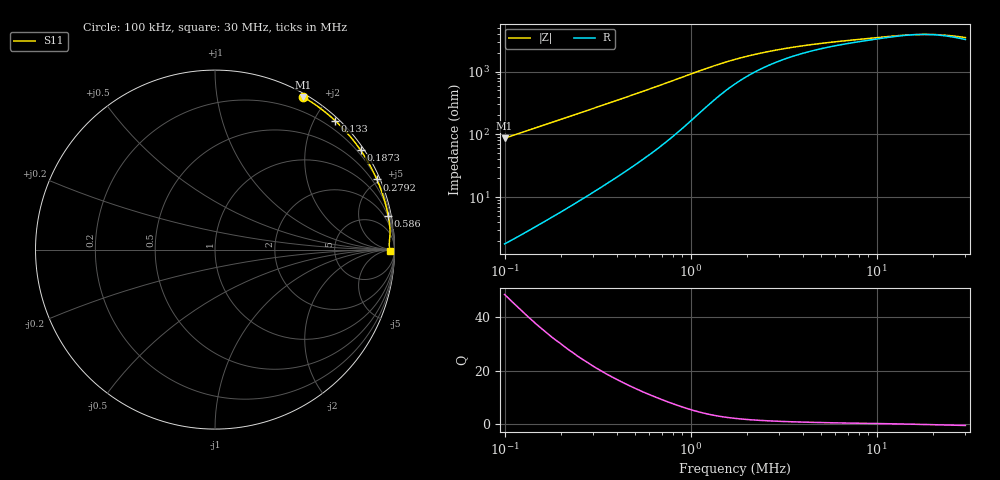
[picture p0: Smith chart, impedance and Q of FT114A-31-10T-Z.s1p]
! ListType=Log
!!FT114A-31 10T Z
# MHz S RI R 50
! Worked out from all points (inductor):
!   101 points, 100 kHz to 30 MHz, reference 50 ohm
!   read as one part to ground: L = 138 uH near 100 kHz
!   highest Q = 48.3 at 100 kHz (marker M1), where L = 138 uH
!   self-resonance near 17.31 MHz
!   S11 on the Smith chart (normalised r, x): 100 kHz: 0.04, +1.73; 133 kHz: 0.06, +2.30; 187.3 kHz: 0.10, +3.23; 279.2 kHz: 0.21, +4.82; 586 kHz: 1, +10; 30 MHz: 65, -25
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0.1  0.4905 0.851
0.1120837  0.5693 0.8002
0.1186625  0.6051 0.7734
0.1330014  0.6695 0.7184
0.140808  0.6982 0.6905
0.1578228  0.7491 0.635
0.1670863  0.7715 0.6077
0.1872765  0.8108 0.5544
0.2099064  0.8434 0.5038
0.2352709  0.8704 0.456
0.2791784  0.9019 0.3906
0.3129135  0.9182 0.3512
0.350725  0.9313 0.3151
0.3931055  0.942 0.2822
0.4406071  0.9505 0.2522
0.4938487  0.9573 0.225
0.5860135  0.965 0.1889
0.6953784  0.9702 0.1578
0.8735868  0.9741 0.1229
1.03662  0.9751 0.1013
1.23008  0.9748 0.0833
1.459644  0.9738 0.0686
1.833715  0.9724 0.0536
2.582017  0.971 0.0378
3.635686  0.9707 0.027
7.631539  0.972 0.0125
15.13097  0.9745 0.00228
30  0.9735 -0.0102
